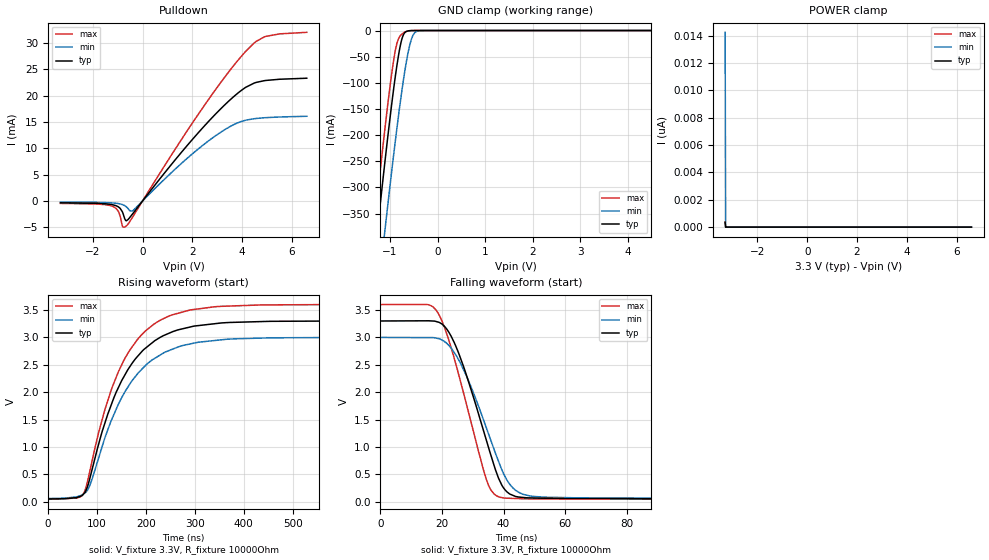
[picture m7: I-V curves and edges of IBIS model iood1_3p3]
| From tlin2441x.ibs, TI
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|   iood1_3p3 Model
[Model]   iood1_3p3
Model_type   I/O_open_drain
Polarity   Non-Inverting
Enable   Active-Low
Vinl = 0.8
Vinh = 2
Vmeas = 1.65
Vref = 3.3
Cref = 2pF
Rref = 10000
|   typ   min   max
C_comp   4.782pF   4.588pF   4.804pF
|  Where Nom  PVT is Nominal Process, 3.3V,   27C
|   Fast PVT is Strong Process,  3.6,   -40C
|   Slow PVT is Weak Process,   3.0V,   150C
[Voltage Range]   3.3   3   3.6
|Junction Temperature
[Temperature Range]   27   150   -40
[Pullup Reference]   3.3   3   3.6
[Pulldown Reference]   0   0   0
[Power Clamp Reference]   3.3   3   3.6
[GND Clamp Reference]   0   0   0
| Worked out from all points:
|   slope of the pulldown table from 0 to 0.495 V, typ, clamps not added: 164 ohm
|   GND clamp passes 1 mA (typ) near -0.63 V on its own axis
|   falling waveform, V_fixture 3.3V, R_fixture 10000Ohm: 20-80 % time 10.9ns typ, 12ns min, 10.1ns max; typ from 3.3 V to 0.053 V
|   rising waveform, V_fixture 3.3V, R_fixture 10000Ohm: 20-80 % time 89.5ns typ, 92.7ns min, 86.7ns max; typ from 0.053 V to 3.3 V
[Pulldown]
|   Voltage   I(typ)   I(min)   I(max)
-3.3V     -352.8uA   -232.8uA   -465.8uA
-1.221V   -699.5uA   -370.9uA   -986.2uA
-993.3mV  -1.064mA   -484uA     -1.825mA
-894.3mV  -1.453mA   -573.1uA   -3.004mA
-815.1mV  -2.036mA   -681.7uA   -4.722mA
-676.5mV  -3.721mA   -1.023mA   -4.835mA
-399.3mV  -2.447mA   -1.872mA   -3.056mA
2.353V    13.57mA    10.33mA    17.26mA
3.373V    18.58mA    13.75mA    23.98mA
4.155V    21.63mA    15.36mA    28.49mA
4.966V    22.92mA    15.84mA    31.31mA
6.6V      23.34mA    16.1mA     32.06mA
[GND Clamp]
|   Voltage   I(typ)   I(min)   I(max)
-3.3V     -2.208A    -2.295A    -2.167A
-1.33V    -437.1mA   -567.1mA   -374mA
-1.231V   -353.3mA   -484.2mA   -289.5mA
-1.102V   -247.4mA   -378.6mA   -184.1mA
-983.4mV  -155mA     -284.1mA   -95.46mA
-884.4mV  -85.51mA   -208.8mA   -36.53mA
-815.1mV  -44.46mA   -158.9mA   -14.45mA
-765.6mV  -21.88mA   -125.3mA   -8.243mA
-666.6mV  -2.381mA   -65.65mA   -2.135mA
-537.9mV  -97.32uA   -13.65mA   -110uA
-359.7mV  -490.2nA   -194.9uA   -171.9nA
6.6V      0A         0A         0A
[POWER Clamp]
|   Voltage   I(typ)   I(min)   I(max)
-3.3V     358.2pA    14.24nA    370.5pA
-3.28V    0A         0A         0A
-3.27V    0A         0A         0A
6.6V      0A         0A         0A
[Ramp]
R_load = 10000
|   typ   min   max
dV/dt_r   1.94827/8.93767e-08   1.76341/9.2347e-08   2.13221/8.6211e-08
dV/dt_f   1.94827/1.08755e-08   1.76341/1.19574e-08   2.13221/1.0091e-08
[Falling Waveform]
V_fixture = 3.3V
V_fixture_min = 3V
V_fixture_max = 3.6V
R_fixture = 10000Ohm
C_fixture = 0F
|   Time   V(typ)   V(min)   V(max)
0s        3.3V       3V         3.6V
15.86ns   3.303V     2.997V     3.593V
18.74ns   3.28V      2.98V      3.443V
21.54ns   3.152V     2.892V     3.064V
27.98ns   2.304V     2.294V     1.774V
35.15ns   986.4mV    1.234V     297.8mV
39.91ns   261.8mV    528.1mV    73.39mV
43.13ns   116.8mV    249.8mV    63.03mV
46.41ns   80.12mV    137.3mV    56.67mV
5us       52.88mV    60.86mV    46.31mV
[Rising Waveform]
V_fixture = 3.3V
V_fixture_min = 3V
V_fixture_max = 3.6V
R_fixture = 10000Ohm
C_fixture = 0F
|   Time   V(typ)   V(min)   V(max)
0s        52.88mV    60.86mV    46.31mV
73.59ns   155mV      152.7mV    170.5mV
85.22ns   429.1mV    300.6mV    562.3mV
103.3ns   1.057V     804.3mV    1.27V
128.7ns   1.763V     1.477V     2.035V
153.8ns   2.268V     1.958V     2.566V
183.1ns   2.657V     2.341V     2.968V
247.2ns   3.077V     2.761V     3.39V
338.6ns   3.248V     2.941V     3.557V
5us       3.3V       3V         3.6V
